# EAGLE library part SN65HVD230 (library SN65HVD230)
Check availability
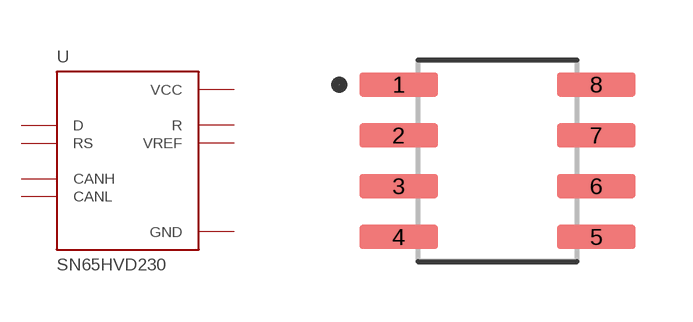
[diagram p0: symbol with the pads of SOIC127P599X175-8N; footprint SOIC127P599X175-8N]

Designator prefix U

## SN65HVD230 (AVAILABILITY: In Stock; CHECK_PRICES: https://www.snapeda.com/parts/SN65HVD230/Texas+Instruments/view-part/?ref=eda; DESCRIPTION: 1/1 Transceiver Half CANbus 8-SOIC; MF: Texas Instruments; MP: SN65HVD230; PACKAGE: SOIC-8 Texas Instruments; PRICE: None; SNAPEDA_LINK: https://www.snapeda.com/parts/SN65HVD230/Texas+Instruments/view-part/?ref=snap)  [SOIC127P599X175-8N]
1  D  in
2  GND  pwr
3  VCC  pwr
4  R  out
5  VREF  out
6  CANL
7  CANH
8  RS  in

## Footprint SOIC127P599X175-8N (pad centres in mm)
smd 1.97 x 0.6: 1 -2.47,1.905; 2 -2.47,0.635; 3 -2.47,-0.635; 4 -2.47,-1.905; 5 2.47,-1.905; 6 2.47,-0.635; 7 2.47,0.635; 8 2.47,1.905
